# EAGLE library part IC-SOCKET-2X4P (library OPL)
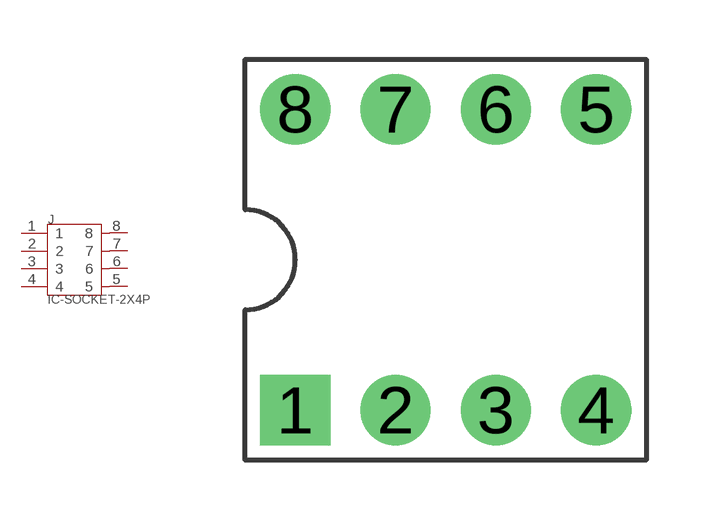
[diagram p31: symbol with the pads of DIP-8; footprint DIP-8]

Designator prefix J

## IC-SOCKET-2X4P-320070014  [DIP-8]
1  1
2  2
3  3
4  4
5  5
6  6
7  7
8  8

## Footprint DIP-8 (pad centres in mm)
drill 1.016 pad 1.778 square: 1 -3.81,-3.81
drill 1.016 pad 1.778: 2 -1.27,-3.81; 3 1.27,-3.81; 4 3.81,-3.81; 5 3.81,3.81; 6 1.27,3.81; 7 -1.27,3.81; 8 -3.81,3.81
